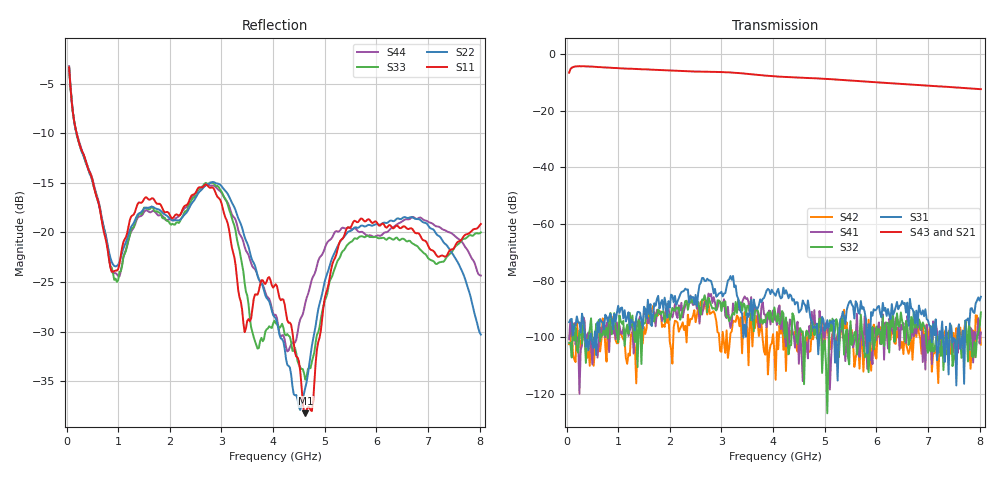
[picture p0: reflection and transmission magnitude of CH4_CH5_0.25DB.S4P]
!Agilent Technologies,E5071C,MY46316741,A.11.02
!Date: Mon Jun 01 11:48:55 2026
!Data & Calibration Information:
!1:CH4 INPUT 2:CH4 OUTPUT 3:CH5 INPUT 4:CH5 OUTPUT
!Freq	S11:SOLT4(ON)	S12:SOLT4(ON)	S13:SOLT4(ON)	S14:SOLT4(ON)
!	S21:SOLT4(ON)	S22:SOLT4(ON)	S23:SOLT4(ON)	S24:SOLT4(ON)
!	S31:SOLT4(ON)	S32:SOLT4(ON)	S33:SOLT4(ON)	S34:SOLT4(ON)
!	S41:SOLT4(ON)	S42:SOLT4(ON)	S43:SOLT4(ON)	S44:SOLT4(ON)
!PortZ  Port1:50+j0  Port2:50+j0  Port3:50+j0  Port4:50+j0
!Above PortZ is port z conversion or system Z0 setting when saving the data.
!When reading, reference impedance value at option line is always used.
# Hz S dB R 50
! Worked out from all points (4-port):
!   320 points, 50 MHz to 8.025 GHz, reference 50 ohm
!   strongest paths, dB at 50 MHz, 2.05 GHz, 4.05 GHz, 6.05 GHz, 8.025 GHz:
!     S43: -6.7, -5.9, -8.0, -10.1, -12.5
!     S21: -6.7, -6.0, -8.2, -10.4, -12.7
!     S31: -94.6, -85.3, -85.3, -88.9, -85.6
!     S32: -101.9, -89.6, -92.1, -97.0, -91.2
!     S41: -100.7, -93.0, -92.8, -94.7, -98.3
!     S42: -102.4, -109.2, -114.9, -99.6, -102.5
!   lowest |S11| = -38.2 dB at 4.625 GHz (marker M1), VSWR 1.02, Z = 51.1 + j0.535 ohm
!   |S11| at or under -10 dB: 196.5 MHz to end of sweep
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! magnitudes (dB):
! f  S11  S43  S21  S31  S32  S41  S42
! 50 MHz  -3.4  -6.7  -6.7  -94.6  -101.9  -100.7  -102.4
! 875 MHz  -23.9  -5.0  -5.1  -93.7  -98.9  -94.6  -92.6
! 2.825 GHz  -15.5  -6.4  -6.5  -81.7  -89.9  -87.8  -91.0
! 4.275 GHz  -28.9  -8.2  -8.4  -84.5  -99.3  -94.7  -96.5
! 4.625 GHz  -38.2  -8.5  -8.7  -88.7  -100.1  -101.4  -101.0
! 5.575 GHz  -18.8  -9.5  -9.7  -93.3  -98.3  -101.5  -110.4
! 8.025 GHz  -19.2  -12.5  -12.7  -85.6  -91.2  -98.3  -102.5
